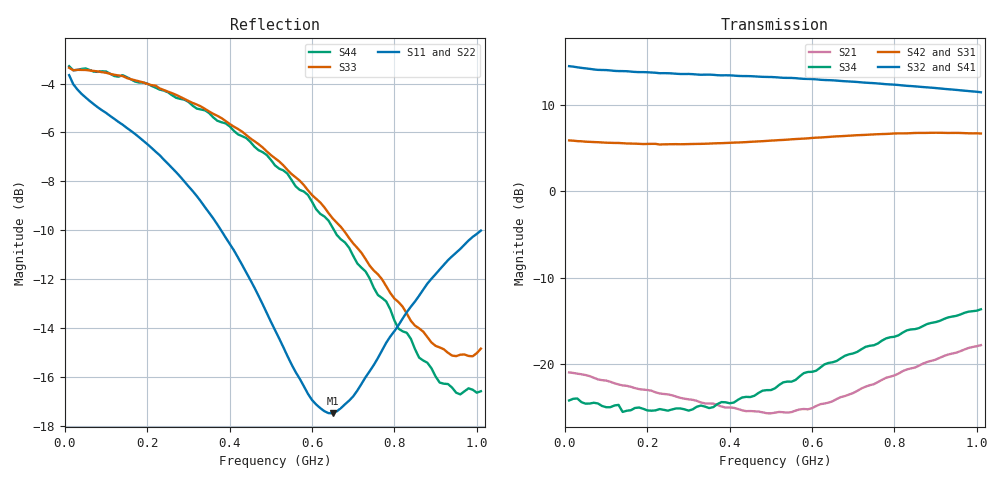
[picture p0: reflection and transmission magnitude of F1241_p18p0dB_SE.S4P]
! Integrated Device Technology
! Corporate Headquarters
! 6024 Silver Creek Valley Road
! San Jose, CA 95138  USA
! Phone:  1-408-284-8200
! Toll Free:  1-800-223-1366
! Webpage:  http://www.idt.com/
! Timing and RF Division
! 515 Groton Road, Suite 102
! Westford, MA 01886-6024
! Device:  F1241
! Description: Dual Intermediate Frequency Digital Variable Gain Amplifier
! Frequency:  10.0 -  500.00 MHz
! Package:  5x5 mm QFN Plastic Package: 32 pin
! Ports:  8 RF, 20 DC
!  Pin  1  = GA3  Pin 17  = RF OUT_B+
!  Pin  2  = GA4  Pin 18  = RF OUT_B-
!  Pin  3  = GA5  Pin 19  = STBY_B
!  Pin  4  = ISET_A  Pin 20  = Ground
!  Pin  5  = ISET_B  Pin 21  = Ground
!  Pin  6  = GB5  Pin 22  = STB_A
!  Pin  7  = GB4  Pin 23  = RF OUT_A-  = Port 4
!  Pin  8  = GB3  Pin 24  = RF OUT_A+  = Port 3
!  Pin  9  = GB2  Pin 25  = NO CONNECT
!  Pin 10  = GB1  Pin 26  = NO CONNECT
!  Pin 11  = RF IN_B+  Pin 27  = VCC
!  Pin 12  = RF IN_B-  Pin 28  = Ground
!  Pin 13  = Ground  Pin 29  = RF IN_A-  = Port 2
!  Pin 14  = VCC  Pin 30  = RF IN_A+  = Port 1
!  Pin 15  = NO CONNECT  Pin 31  = GA1
!  Pin 16  = NO CONNECT  Pin 32  = GA2
! State:  2
! Gain State:  18.0 dB
! Voltages:  Vcc = +5.00 Volts  Icc approximately 160.0 mA or 80 mA per channel.
! Data:  The device was measured on a custom evaluation board which has
!  individual transmission lines to the RF pins.  Data was collected
!  using a calibrated network analyzer.  The evaluation board was
!  de-embedded using a port reference technique.
!  The reference plane is the edge of the package pin.
!  Only Channel A was measured.
!  This data is in single-ended operation.  If your needs are balanced
!  or differential S-parameters then this file needs to be used a
!  linear simulator.
! Misc:  Lot Code  160028MY
!  Action Tracker AT004
! Date Measured:  2014-08-14
! Date:  2014-08-28  MJV
! Note:
!  Integrated Device Technology supplies this data as a sample of measured
!  data at the package pin for this product.  Your particular data for this
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# Hz S dB R 50
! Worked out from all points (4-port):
!   101 points, 10 MHz to 1.01 GHz, reference 50 ohm
!   strongest paths, dB at 10 MHz, 260 MHz, 510 MHz, 760 MHz, 1.01 GHz:
!     S32: 14.5, 13.7, 13.2, 12.5, 11.5
!     S41: 14.5, 13.6, 13.1, 12.3, 11.2
!     S42: 5.9, 5.5, 5.9, 6.6, 6.7
!     S31: 5.9, 5.4, 5.6, 6.3, 6.5
!     S34: -24.2, -25.2, -22.8, -17.6, -13.6
!     S21: -21.0, -23.6, -25.6, -22.1, -17.8
!   lowest |S11| = -17.5 dB at 650 MHz (marker M1), VSWR 1.31, Z = 39.5 - j5.78 ohm
!   |S11| at or under -10 dB: 379 MHz to end of sweep
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1e7  -3.65 -9.9  -20.96 7.2  -49.35 37.7  -24.58 5.5
     -20.96 7.1  -3.66 -9.7  -24.59 5.1  -49.41 37.5
     5.91 4.4  14.52 -174.5  -3.35 -6.3  -24.21 16.0
     14.53 -174.4  5.91 4.6  -24.14 15.2  -3.29 -6.5
5e7  -4.57 -12.9  -21.34 -12.0  -43.85 56.2  -24.94 -2.7
     -21.27 -11.9  -4.60 -12.5  -24.89 -2.6  -44.10 57.7
     5.79 -5.4  14.26 172.7  -3.44 -5.1  -24.58 -9.4
     14.26 172.3  5.77 -5.3  -24.35 -8.0  -3.38 -5.2
2.6e8  -7.45 -39.5  -23.67 -51.0  -31.26 54.9  -24.84 -5.9
       -23.61 -53.5  -7.40 -37.6  -24.86 -6.1  -31.30 54.5
       5.35 -25.8  13.68 145.3  -4.39 -20.6  -25.25 -62.1
       13.60 144.6  5.48 -25.4  -26.06 -60.7  -4.47 -19.9
4.7e8  -12.68 -75.5  -25.94 -105.5  -26.63 35.0  -23.73 -14.6
       -25.49 -111.3  -12.68 -72.0  -23.59 -14.3  -26.57 34.2
       5.50 -43.4  13.30 119.8  -6.48 -37.1  -23.33 -124.8
       13.17 118.7  5.80 -44.1  -26.06 -135.2  -6.72 -34.8
6.5e8  -17.49 -147.4  -24.97 -172.5  -24.50 17.0  -22.99 -27.4
       -24.30 -177.6  -17.85 -144.4  -22.74 -27.5  -24.35 15.2
       6.04 -60.9  12.88 97.5  -9.51 -55.2  -19.78 -177.9
       12.67 96.5  6.36 -62.9  -21.73 168.9  -9.89 -51.3
8.1e8  -13.89 154.9  -21.81 140.2  -23.45 1.5  -22.93 -41.2
       -21.09 137.1  -14.08 155.5  -22.52 -41.3  -23.26 -0.8
       6.45 -79.8  12.33 77.9  -12.94 -78.8  -16.66 146.2
       12.09 77.0  6.73 -82.7  -17.48 130.8  -14.03 -72.6
1.01e9  -10.02 129.7  -18.21 101.5  -22.71 -15.8  -23.63 -57.9
        -17.80 98.5  -10.11 131.1  -23.07 -58.0  -22.50 -18.9
        6.47 -106.9  11.49 53.6  -14.85 -132.6  -13.65 107.7
        11.22 52.9  6.72 -110.3  -14.04 94.2  -16.59 -131.2
